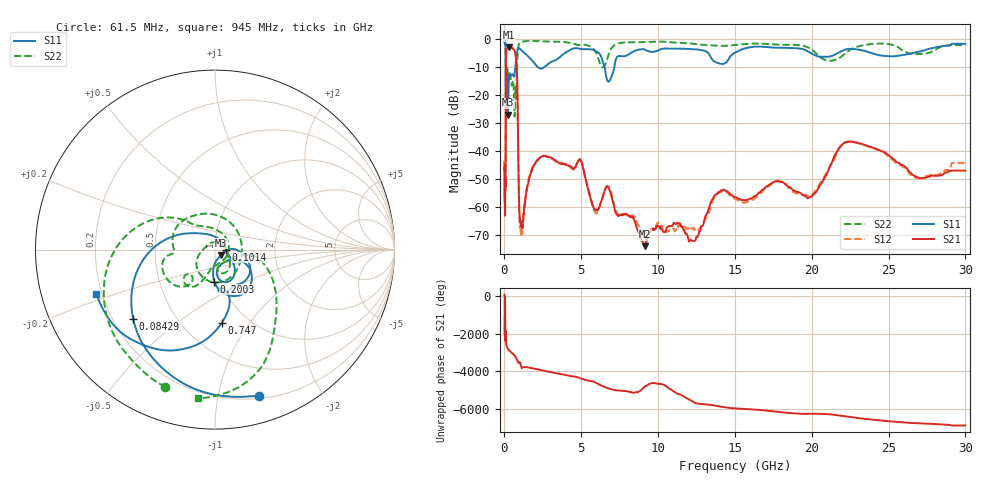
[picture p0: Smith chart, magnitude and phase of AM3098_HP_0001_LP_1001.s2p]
! Date/Time: Thu, Feb 28, 2019 8:32 AM
! Network Analyzer: Agilent Technologies E8364B Rev: A.07.50.67
! Sweep from 0.010 to 30.000 GHz, 1601 Points, Sweep Type: LOG
! Power Supply: 5.023 V, 0.002 A
# Hz S DB R 50
!freq MagS11 AngS11 MagS21 AngS21 MagS12 AngS12 MagS22 AngS22
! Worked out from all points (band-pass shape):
!   1601 points, 10 MHz to 30 GHz, reference 50 ohm
!   highest |S21| = -2.77 dB at 266.5 MHz (marker M1); lowest = -73.9 dB at 9.118 GHz (marker M2)
!   |S21| within 3 dB of the highest: 105.6 MHz to 734.9 MHz (629.3 MHz wide, 150 % of centre)
!   lowest |S11| = -26.9 dB at 233.9 MHz (marker M3), VSWR 1.10, Z = 53.5 - j3.16 ohm
!   |S11| at or under -10 dB: 91.05 MHz to 701.6 MHz (610.6 MHz wide, 154 % of centre); 2.194 GHz to 2.546 GHz (352.9 MHz wide, 14.9 % of centre); 6.524 GHz to 7.148 GHz (623.7 MHz wide, 9.12 % of centre)
!   |S22| runs from -27.6 to -0.5 dB; largest |S21 - S12| = 0.012
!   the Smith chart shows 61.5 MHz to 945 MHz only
!   S11 on the Smith chart (normalised r, x): 61.5 MHz: 0.22, -1.32; 84.29 MHz: 0.28, -0.34; 101.4 MHz: 1.13, -0.00; 200.3 MHz: 0.93, -0.34; 747 MHz: 0.76, -0.75; 945 MHz: 0.18, -0.18
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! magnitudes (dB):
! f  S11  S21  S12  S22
! 10 MHz  -0.3  -46.5  -43.9  -0.6
! 38.04 MHz  -0.5  -60.8  -58.6  -1.0
! 61.5 MHz  -1.4  -51.9  -52.8  -1.8
! 74.38 MHz  -2.3  -47.8  -49.3  -2.7
! 84.29 MHz  -4.5  -29.3  -29.4  -4.9
! 101.4 MHz  -24.2  -6.7  -6.7  -16.7
! 144.7 MHz  -14.7  -3.4  -3.4  -12.8
! 200.3 MHz  -15.0  -3.1  -3.1  -10.9
! 233.9 MHz  -26.9  -2.8  -2.8  -12.5
! 266.5 MHz  -17.4  -2.8  -2.7  -12.9
! 550.5 MHz  -12.5  -3.3  -3.3  -14.7
! 747 MHz  -7.7  -6.3  -6.2  -21.0
! 833.9 MHz  -4.2  -15.9  -15.9  -7.6
! 945 MHz  -3.0  -57.3  -57.4  -1.6
! 1.126 GHz  -3.9  -66.7  -68.3  -0.8
! 2.084 GHz  -9.4  -43.5  -43.5  -0.6
! 4.903 GHz  -3.3  -42.7  -42.8  -2.0
! 7.926 GHz  -5.8  -62.4  -62.8  -1.0
! 9.118 GHz  -3.6  -73.9  -71.0  -0.9
! 19.7 GHz  -4.1  -56.8  -55.7  -2.7
! 22.67 GHz  -3.4  -36.6  -36.6  -3.2
! 30 GHz  -1.5  -46.9  -44.1  -2.0
